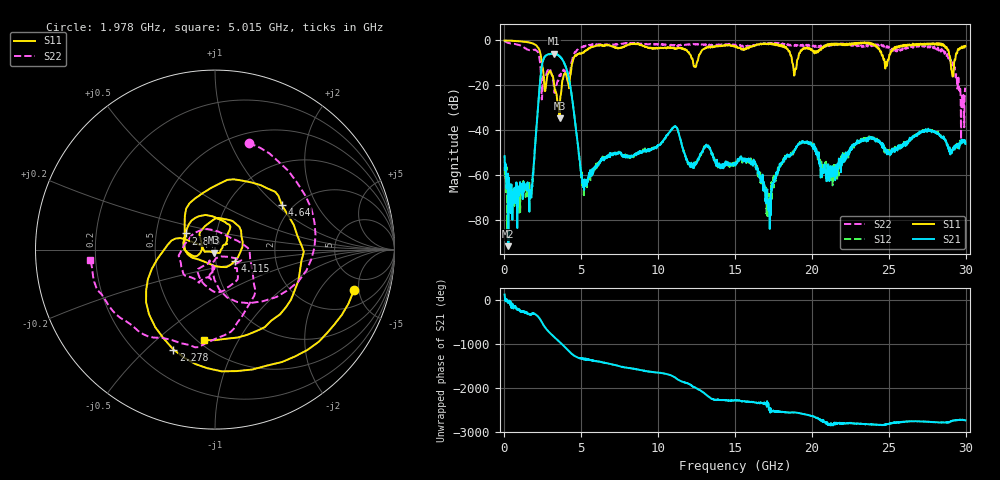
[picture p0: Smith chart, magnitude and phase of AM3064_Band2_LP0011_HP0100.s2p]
# Hz S DB R 50.0
!freq dBS11 angS11 dBS21 angS21 dBS12 angS12 dBS22 angS22
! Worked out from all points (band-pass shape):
!   1600 points, 10 MHz to 29.98 GHz, reference 50 ohm
!   highest |S21| = -5.87 dB at 3.234 GHz (marker M1); lowest = -91.9 dB at 253.7 MHz (marker M2)
!   |S21| within 3 dB of the highest: 2.52 GHz to 3.795 GHz (1.275 GHz wide, 40.4 % of centre)
!   lowest |S11| = -34.8 dB at 3.59 GHz (marker M3), VSWR 1.04, Z = 49.2 - j1.62 ohm
!   |S11| at or under -10 dB: 2.433 GHz to 4.426 GHz (1.992 GHz wide, 58.1 % of centre); 12.27 GHz to 12.52 GHz (242 MHz wide, 1.95 % of centre); 18.72 GHz to 19.02 GHz (296.2 MHz wide, 1.57 % of centre)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
!   |S22| runs from -44.2 to -0.2 dB; largest |S21 - S12| = 0.012
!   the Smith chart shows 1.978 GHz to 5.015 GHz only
!   S11 on the Smith chart (normalised r, x): 1.978 GHz: 3.44, -4.44; 2.278 GHz: 0.35, -0.61; 2.878 GHz: 0.71, +0.13; 4.115 GHz: 1.24, -0.16; 4.64 GHz: 1.76, +1.09; 5.015 GHz: 0.54, -0.73
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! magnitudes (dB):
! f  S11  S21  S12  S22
! 10 MHz  -0.1  -51.7  -56.7  -0.2
! 253.7 MHz  -0.1  -91.9  -71.8  -1.2
! 1.678 GHz  -1.1  -68.2  -71.5  -4.4
! 1.978 GHz  -1.9  -48.6  -48.2  -4.1
! 2.278 GHz  -4.4  -21.5  -21.6  -8.1
! 2.878 GHz  -14.6  -6.2  -6.2  -12.7
! 3.234 GHz  -20.0  -5.9  -6.0  -22.4
! 3.59 GHz  -34.8  -7.1  -7.2  -15.3
! 4.115 GHz  -17.8  -14.8  -14.7  -18.3
! 4.64 GHz  -7.0  -38.9  -38.8  -5.1
! 5.015 GHz  -5.9  -59.9  -58.7  -3.1
! 10 GHz  -3.5  -47.3  -46.8  -1.8
! 15 GHz  -2.6  -55.9  -54.6  -1.9
! 16.34 GHz  -2.2  -55.5  -56.9  -2.2
! 17.16 GHz  -1.6  -75.6  -73.7  -1.4
! 18.27 GHz  -3.2  -51.7  -52.3  -2.0
! 19.99 GHz  -4.2  -46.7  -47.2  -2.1
! 21.27 GHz  -1.5  -57.4  -57.9  -2.0
! 25 GHz  -8.3  -50.7  -49.5  -2.8
! 28.56 GHz  -2.2  -42.9  -42.9  -4.6
! 29.16 GHz  -16.2  -48.9  -48.7  -9.8
! 29.98 GHz  -2.5  -46.3  -45.7  -21.7
